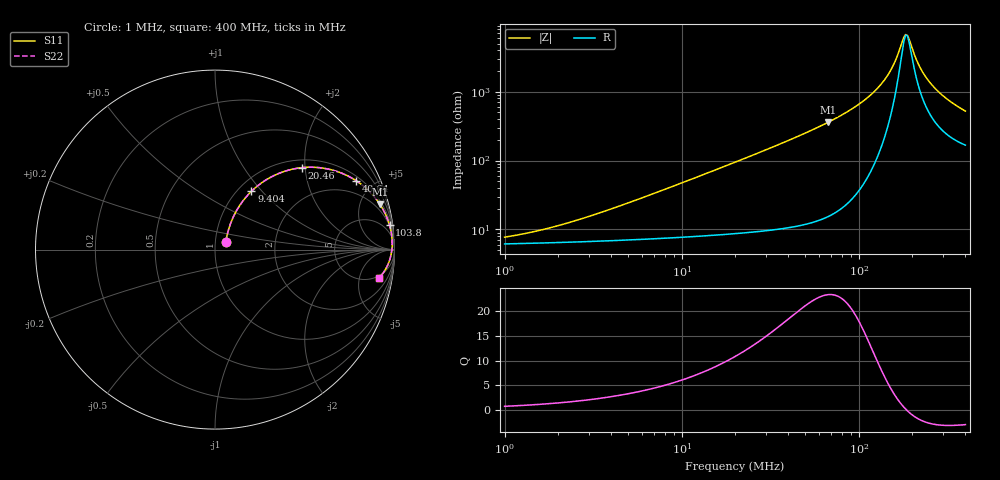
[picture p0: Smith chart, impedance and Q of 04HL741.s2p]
! Coilcraft 0402HL-741 Chip Inductor
! 20 July 2012
# MHz S MA R 50
!Freq  MagS11  AngS11  MagS21  AngS21  MagS12  AngS12  MagS22  AngS22
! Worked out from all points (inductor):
!   263 points, 1 MHz to 400 MHz, reference 50 ohm
!   read as one part in series: L = 740 nH near 4.524 MHz
!   highest Q = 23.4 at 67.2 MHz (marker M1), where L = 852 nH
!   self-resonance near 183.8 MHz
!   S11 on the Smith chart (normalised r, x): 1 MHz: 1.12, +0.09; 9.404 MHz: 1.15, +0.88; 20.46 MHz: 1.17, +1.93; 40.64 MHz: 1.21, +3.97; 103.8 MHz: 2, +14; 400 MHz: 4, -10
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1  0.07256 34.6  0.9412 -2.5  0.9412 -2.5  0.07256 34.6
2.735188  0.1335 55.7  0.9314 -6.8  0.9314 -6.8  0.1335 55.7
7.481253  0.3155 60.1  0.8859 -18.0  0.8859 -18.0  0.3155 60.1
9.403502  0.3829 58.0  0.8606 -22.2  0.8606 -22.2  0.3829 58.0
13.55795  0.51 52.4  0.7983 -30.4  0.7983 -30.4  0.51 52.4
20  0.6573 43.8  0.6957 -40.9  0.6957 -40.9  0.6573 43.8
20.46263  0.6659 43.3  0.6885 -41.5  0.6885 -41.5  0.6659 43.3
28.18402  0.7769 35.2  0.5777 -50.8  0.5777 -50.8  0.7769 35.2
40.63566  0.8747 26.1  0.4401 -60.9  0.4401 -60.9  0.8747 26.1
54.70376  0.9281 19.4  0.3328 -68.0  0.3328 -68.0  0.9281 19.4
67.2049  0.9531 15.3  0.2647 -72.2  0.2647 -72.2  0.9531 15.3
103.7767  0.982 8.0  0.1398 -78.6  0.1398 -78.6  0.982 8.0
127.4922  0.9872 5.0  0.0883 -79.2  0.0883 -79.2  0.9872 5.0
149.6251  0.9882 2.9  0.05098 -75.2  0.05098 -75.2  0.9882 2.9
163.9572  0.9877 1.7  0.0312 -65.9  0.0312 -65.9  0.9877 1.7
179.6621  0.9862 0.5  0.01594 -30.1  0.01594 -30.1  0.9862 0.5
183.818  0.9857 0.2  0.01455 -11.6  0.01455 -11.6  0.9857 0.2
188.07  0.9852 -0.1  0.01495 8.2  0.01495 8.2  0.9852 -0.1
215.7291  0.9807 -1.9  0.03769 58.3  0.03769 58.3  0.9807 -1.9
247.456  0.974 -3.6  0.06746 65.6  0.06746 65.6  0.974 -3.6
304.0057  0.9591 -6.2  0.114 65.9  0.114 65.9  0.9591 -6.2
400  0.9287 -9.7  0.1779 61.6  0.1779 61.6  0.9287 -9.7
